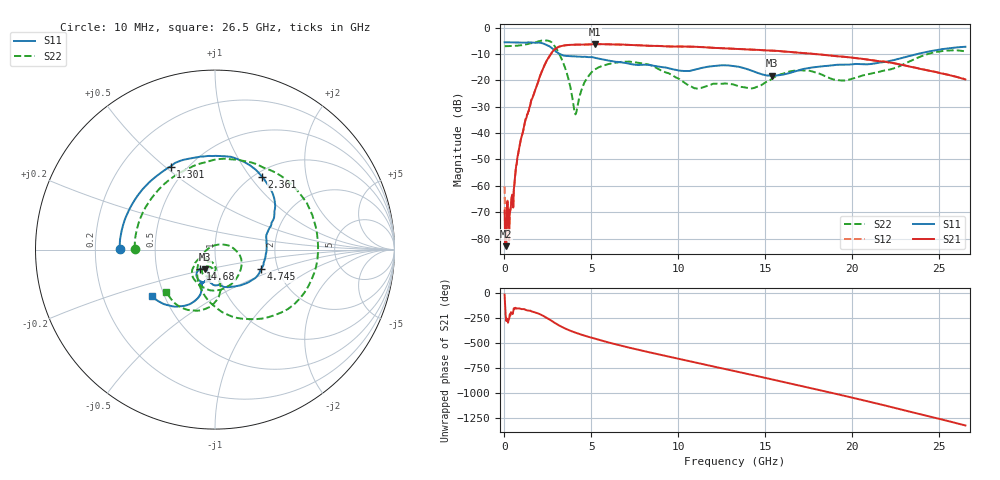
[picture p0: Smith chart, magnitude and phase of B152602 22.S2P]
!  2-Port S-parameters saved by WinCal
! VAR MeasName=S-Parameters (CALIBRATED_DATA) read from VNA (N5242A)
! VAR MeasDate=2016-1-5 16:28:29
! VAR NAME=B152602 22
! VAR FILENAME=B152602 22.S2P
! VAR DATE=2016-1-5 16:28:29
! VAR PHYS_PORTS=1,2
# Hz S DB R 50
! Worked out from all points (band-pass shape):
!   801 points, 10 MHz to 26.5 GHz, reference 50 ohm
!   highest |S21| = -6.19 dB at 5.209 GHz (marker M1); lowest = -82.9 dB at 109.3 MHz (marker M2)
!   |S21| within 3 dB of the highest: 2.745 GHz to 16.48 GHz (13.74 GHz wide, 143 % of centre)
!   lowest |S11| = -18.2 dB at 15.37 GHz (marker M3), VSWR 1.28, Z = 43.6 - j9.68 ohm
!   |S11| at or under -10 dB: 3.203 GHz to 23.71 GHz (20.51 GHz wide, 152 % of centre)
!   |S22| runs from -32.9 to -4.8 dB; largest |S21 - S12| = 0.0032
!   S11 on the Smith chart (normalised r, x): 10 MHz: 0.31, +0.00; 1.301 GHz: 0.41, +0.52; 2.361 GHz: 1.08, +1.14; 4.745 GHz: 1.64, -0.38; 14.68 GHz: 0.83, -0.18; 26.5 GHz: 0.43, -0.27
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1e7  -5.50 179.4  -69.47 -17.3  -60.28 -114.2  -6.97 179.4
1.093375e8  -5.48 174.8  -82.91 77.6  -79.49 65.3  -6.96 173.4
1.755625e8  -5.50 171.5  -65.93 84.3  -65.65 82.3  -6.95 169.2
4.0735e8  -5.53 160.5  -65.00 159.6  -64.35 151.6  -6.91 154.9
8.047e8  -5.60 141.8  -47.42 -155.5  -47.41 -156.1  -6.74 130.2
1.301388e9  -5.60 118.1  -32.88 -175.0  -32.89 -175.2  -6.23 97.6
2.360988e9  -6.33 57.1  -13.36 117.2  -13.36 117.2  -4.81 5.5
2.9239e9  -8.81 26.9  -8.01 56.7  -8.01 56.7  -7.30 -63.8
4.049725e9  -10.84 -1.3  -6.41 -35.3  -6.40 -35.3  -32.44 128.8
4.447075e9  -11.02 -13.5  -6.39 -58.9  -6.38 -58.8  -23.32 21.7
4.745088e9  -11.07 -22.8  -6.34 -74.6  -6.33 -74.6  -19.19 0.7
5.208662e9  -11.40 -38.3  -6.19 -98.3  -6.18 -98.2  -15.75 -25.2
6.8974e9  -13.28 -74.3  -6.41 -175.5  -6.40 -175.4  -12.86 -87.4
8.851038e9  -14.72 -98.7  -6.89 106.2  -6.86 106.1  -15.65 -139.3
1.116891e10  -15.52 -99.4  -7.28 17.1  -7.25 17.2  -22.92 -128.9
1.3255e10  -14.62 -121.5  -7.96 -61.9  -7.95 -62.1  -21.68 -121.8
1.467884e10  -17.40 -127.5  -8.43 -116.4  -8.40 -116.4  -22.03 -94.3
1.53742e10  -18.20 -117.4  -8.68 -143.2  -8.65 -143.2  -19.41 -87.6
1.769208e10  -15.06 -105.8  -9.87 125.7  -9.83 125.8  -16.56 -118.4
2.01424e10  -13.77 -112.4  -11.45 27.8  -11.43 27.8  -19.05 -94.7
2.209604e10  -12.66 -108.5  -13.14 -53.6  -13.08 -53.8  -15.94 -85.8
2.65e10  -7.20 -143.6  -19.61 116.8  -19.58 116.4  -8.92 -139.1
